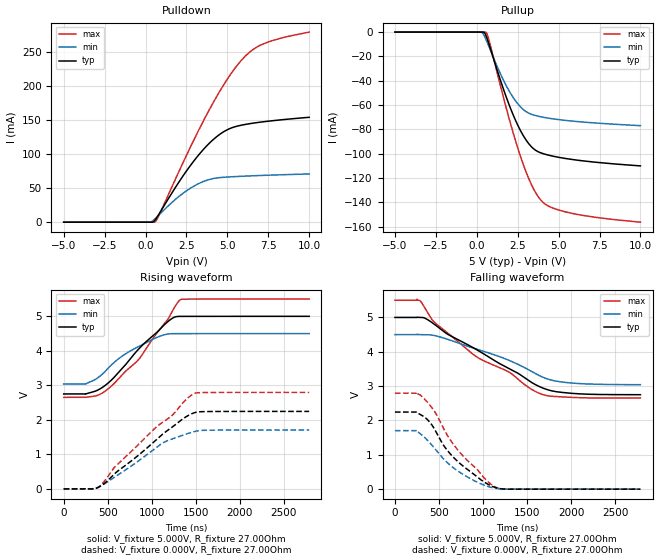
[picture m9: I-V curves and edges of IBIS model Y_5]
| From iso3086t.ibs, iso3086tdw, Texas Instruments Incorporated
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|   Y_5 Model
[Model]   Y_5
Model_type   Output
|Signals   Y   positive pin
Polarity   Non-Inverting
Enable   Active-Low
Vmeas   = 2.5
Vref   = 2.5
Cref   = 50pF
Rref = 27   |Note: 54 Ohm differential load;
Rref_diff   = 54
Cref_diff   = 7pF
| C_comp   obtained at 20MHz
|   typ   min   max
|3-state   Slow PVT   Nom PVT   Fast PVT
C_comp   15.839074pF  15.838838pF   17.853428pF
|High   Nom PVT   Fast PVT   Slow PVT
|C_comp   18.732595pF  17.232594pF   22.191304pF
|Low   Nom PVT   Fast PVT   Slow PVT
|C_comp   18.364210pF  17.392850pF   20.781923pF
[Model Spec]
Vmeas   2.5V   2.25V   2.75V
Vref   2.5V   2.25V   2.75V
[Voltage Range]   5   4.5   5.5
[Temperature Range]   40   125   -40
[Pullup Reference]   5   4.5   5.5
[Pulldown Reference]   0   0   0
[Power Clamp Reference]   5   4.5   5.5
[GND Clamp Reference]   0   0   0
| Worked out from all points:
|   slope of the pulldown table from 0 to 0.75 V, typ, clamps not added: 82.5 ohm
|   slope of the pullup table from 0 to 0.75 V, typ, clamps not added: 74.5 ohm
|   falling waveform, V_fixture 5.000V, R_fixture 27.00Ohm: 20-80 % time 920ns typ, 846ns min, 966ns max; typ from 5 V to 2.75 V
|   rising waveform, V_fixture 5.000V, R_fixture 27.00Ohm: 20-80 % time 505ns typ, 471ns min, 553ns max; typ from 2.75 V to 5 V
|   rising waveform, V_fixture 0.000V, R_fixture 27.00Ohm: 20-80 % time 652ns typ, 574ns min, 715ns max; typ from 0 V to 2.25 V
|   falling waveform, V_fixture 0.000V, R_fixture 27.00Ohm: 20-80 % time 450ns typ, 441ns min, 483ns max; typ from 2.25 V to 0 V
[Pulldown]
|   Voltage   I(typ)   I(min)   I(max)
-5V       -22.04fA   -92.29fA   -8.571fA
212.5mV   268.2nA    28.3uA     135.1nA
580mV     3.082mA    4.901mA    398.4uA
925mV     15.87mA    13.09mA    15.31mA
2.147V    62.68mA    39.7mA     79.76mA
3.475V    104.9mA    59.01mA    145.5mA
4.585V    129.6mA    65.44mA    193.9mA
5.688V    141.3mA    67.09mA    232.5mA
6.475V    144.8mA    67.94mA    251.4mA
7.143V    147mA      68.56mA    260.8mA
8.29V     150.1mA    69.5mA     269.8mA
10V       153.8mA    70.71mA    278.7mA
[Pullup]
|   Voltage   I(typ)   I(min)   I(max)
-5V       141.9fA    51.55fA    282.4fA
205mV     -613nA     -23.85uA   -503.5nA
377.5mV   -33.72uA   -1.141mA   -598.7nA
572.5mV   -3.105mA   -6.301mA   -308.7uA
797.5mV   -12.07mA   -13.69mA   -9.251mA
1.615V    -46.33mA   -39.13mA   -52.95mA
2.402V    -73.62mA   -57.21mA   -90.92mA
3.19V     -92.05mA   -66.78mA   -120.9mA
3.91V     -99.36mA   -69.66mA   -138.2mA
4.487V    -101.6mA   -71.05mA   -143.9mA
5.673V    -104.5mA   -73.03mA   -148.7mA
10V       -110.1mA   -77.02mA   -156.4mA
[Ramp]
R_load = 27.00Ohm
|   typ   min   max
dV/dt_r   1.347V/652.382ns   1.023V/573.942ns   1.678V/715.394ns
dV/dt_f   1.350V/920.107ns 874.975mV/845.900ns   1.709V/966.353ns
[Falling Waveform]
V_fixture = 5.000V
V_fixture_min = 4.500V
V_fixture_max = 5.500V
R_fixture = 27.00Ohm
|   Time   V(typ)   V(min)   V(max)
0s        5V         4.5V       5.5V
285ns     5.002V     4.502V     5.49V
437.5ns   4.821V     4.479V     4.887V
597.5ns   4.513V     4.365V     4.55V
885ns     4.124V     4.112V     3.932V
1.295us   3.515V     3.751V     3.408V
1.507us   3.18V      3.491V     2.98V
1.645us   2.982V     3.299V     2.786V
1.992us   2.794V     3.093V     2.674V
2.787us   2.751V     3.042V     2.652V
[Rising Waveform]
V_fixture = 5.000V
V_fixture_min = 4.500V
V_fixture_max = 5.500V
R_fixture = 27.00Ohm
|   Time   V(typ)   V(min)   V(max)
0s        2.751V     3.042V     2.652V
252.5ns   2.754V     3.043V     2.653V
390ns     2.866V     3.222V     2.715V
512.5ns   3.084V     3.515V     2.914V
665ns     3.493V     3.849V     3.308V
860ns     4.076V     4.136V     3.777V
1.205us   4.893V     4.493V     5.012V
1.285us   4.993V     4.498V     5.367V
1.33us    4.998V     4.499V     5.487V
2.787us   5V         4.5V       5.5V
[Rising Waveform]
V_fixture = 0.000V
V_fixture_min = 0.000V
V_fixture_max = 0.000V
R_fixture = 27.00Ohm
|   Time   V(typ)   V(min)   V(max)
0s        -8.474uV   -22.69uV   -9.652uV
340ns     2.441mV    8.032mV    -29.94uV
397.5ns   49.97mV    55.45mV    56.75mV
465ns     166.3mV    147.8mV    231mV
577.5ns   437mV      343.5mV    627.5mV
1.125us   1.588V     1.33V      1.932V
1.24us    1.805V     1.455V     2.151V
1.363us   2.046V     1.565V     2.518V
1.485us   2.208V     1.662V     2.767V
2.787us   2.245V     1.705V     2.796V
[Falling Waveform]
V_fixture = 0.000V
V_fixture_min = 0.000V
V_fixture_max = 0.000V
R_fixture = 27.00Ohm
|   Time   V(typ)   V(min)   V(max)
0s        2.245V     1.705V     2.796V
252.5ns   2.227V     1.714V     2.783V
305ns     2.151V     1.579V     2.705V
382.5ns   1.99V      1.389V     2.491V
450ns     1.746V     1.189V     2.261V
557.5ns   1.258V     865.4mV    1.736V
692.5ns   855.7mV    568mV      1.209V
995ns     238.8mV    135.3mV    381.9mV
1.163us   32.09mV    16.55mV    35.44mV
2.787us   -8.474uV   -22.69uV   -9.652uV
